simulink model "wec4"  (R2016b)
settings: Solver=ode4  StartTime=0  StopTime=1000  FixedStep=0.005  MaxStep=0.005  RelTol=1e-3  EnableMultiTasking=on
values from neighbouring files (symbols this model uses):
  arAdaptiveLawData = 1/2*zModelSimple.zModelPto.arFreq.*     zModelSimple.zModelPto.arMagnitude./     cos(zModelSimple.zModelPto.arPhase*pi/180+pi/2)    [IMPACT_Control.m]
  arAdaptiveLawDataX = 1/2*zModelSimpleX.zModelPto.arFreq.*         zModelSimpleX.zModelPto.arMagnitude./         cos(zModelSimpleX.zModelPto.arPhase*pi/180+pi/2)    [IMPACT_Control.m]
  arControllerRampGain = [0,0,1,1]    [IMPACT_Control.m]
  arControllerRampTime = [0 rStartRampTime rStartRampTime+rRampTimeLength 8000]    [IMPACT_Control.m]
  arEkfInitialisation = zeros(1,11)    [IMPACT_Control.m]
  arEkfInitialisationX = zeros(1,11)    [IMPACT_Control.m]
  arFrequency = zModelSimple.zModelPto.arFreq    [IMPACT_Control.m]
  arFrequencyRange = zModelSimple.zModelPto.arFreq    [IMPACT_Control.m]
  arFrequencyX = zModelSimpleX.zModelPto.arFreq    [IMPACT_Control.m]
  arImpedance = 1./zModelSimple.zModelPto.arMagnitude./zModelSimple.zModelPto.arFreq    [IMPACT_Control.m]
  arImpedanceX = 1./zModelSimpleX.zModelPto.arMagnitude./zModelSimpleX.zModelPto.arFreq    [IMPACT_Control.m]
  CentralPTOPreload = -1.6113e+07    (= -16113000)    [wecSimInputFile.m]
  F1 = [4.243 2.375 -12.243]    [wecSimInputFile.m]
  F2 = [4.243 -2.375 -12.243]    [wecSimInputFile.m]
  F3 = [-4.243 -2.375 -12.243]    [wecSimInputFile.m]
  F4 = [-4.243 2.375 -12.243]    [wecSimInputFile.m]
  FC = [0 0 -14]    [wecSimInputFile.m]
  iAdaptiveDamping = 0    [wec4IMPACT_Project.m]    (also in IMPACT_Control.m = handles.iAdaptiveDamping; wec1_IMPACT_Project.m; wec2_IMPACT_Project.m; wec3_IMPACT_Project.m)
  iControlType = 2    [wec4IMPACT_Project.m]    (also in IMPACT_Control.m = handles.iControlType; wec1_IMPACT_Project.m = 1; wec2_IMPACT_Project.m = 1; wec3_IMPACT_Project.m = 1)
  iPtoPositionConstraint = 1    [wec4IMPACT_Project.m]    (also in IMPACT_Control.m = handles.iPtoPositionConstraint; wec1_IMPACT_Project.m = 0; wec2_IMPACT_Project.m; wec3_IMPACT_Project.m)
  iSensorNoise = 0    [IMPACT_Control.m]
  m = m+1    (= 2)    [checkParamFile.m]
  PTOrotation = atan((T1(2)-F1(2))/(T1(1)-F1(1)))    [wecSimInputFile.m]
  rCogFloater = -8    [wec4_IMPACT_Model.m]    (also in paramInitial.m = get( handles.edit_rCogFloater, 'String' ); wec1_IMPACT_Model.m = -18; wec2_IMPACT_Model.m = -8.5; wec3_IMPACT_Model.m = -0.7)
  rCogSpar = -36.6    [wec4_IMPACT_Model.m]    (also in paramInitial.m = get( handles.edit_rCogSpar, 'String' ); wec3_IMPACT_Model.m = -21.3; wec3_IMPACT_Model2.m = -21.3)
  rDisplacementLimit = 10.000000    (= 10)    [wec4IMPACT_Project.m]    (also in IMPACT_Control.m = getValue(handles.edit_displacementLimit); wec1_IMPACT_Project.m; wec2_IMPACT_Project.m; wec3_IMPACT_Project.m = 3)
  rDisplacementLimitX = 10.000000    (= 10)    [wec4IMPACT_Project.m]    (also in IMPACT_Control.m = getValue(handles.edit_displacementLimitX); wec1_IMPACT_Project.m = 0; wec2_IMPACT_Project.m; wec3_IMPACT_Project.m = 0)
  rGainForAntiWIndUp = tfControllerDiscrete.rGain    [IMPACT_Control.m]
  rGainForAntiWIndUpX = tfControllerXDiscrete.rGain    [IMPACT_Control.m]
  rMaxForcePto = 300000000.000000    (= 300000000)    [wec4IMPACT_Project.m]    (also in IMPACT_Control.m = getValue(handles.edit_maxForcePto); wec1_IMPACT_Project.m = 1e+15; wec2_IMPACT_Project.m = 1e+15; wec3_IMPACT_Project.m = 1000000000)
  rMinForcePto = -300000000.000000    (= -300000000)    [wec4IMPACT_Project.m]    (also in IMPACT_Control.m = getValue(handles.edit_minForcePto); wec1_IMPACT_Project.m = -1e+15; wec2_IMPACT_Project.m = -1e+15; wec3_IMPACT_Project.m = -1000000000)
  rMooringX = 20000    [wec4_IMPACT_Model.m]    (also in paramInitial.m = get( handles.edit_rMooringX, 'String' ); wec3_IMPACT_Model.m = 10000; wec3_IMPACT_Model2.m = 10000)
  rMooringZ = 10000    [wec4_IMPACT_Model.m]    (also in paramInitial.m = get( handles.edit_rMooringZ, 'String' ); wec3_IMPACT_Model.m = 0; wec3_IMPACT_Model2.m = 0)
  rOutputSampleTime = 0.010000    (= 0.01)    [wec4IMPACT_Project.m]    (also in IMPACT_Control.m = getValue(handles.edit_outputSampleTime); wec1_IMPACT_Project.m; wec2_IMPACT_Project.m; wec3_IMPACT_Project.m)
  rPassiveDampingGain = -604830.000000    (= -604830)    [wec4IMPACT_Project.m]    (also in IMPACT_Control.m = getValue(handles.edit_gainPLD); wec1_IMPACT_Project.m = -214018.1537; wec2_IMPACT_Project.m = -1948070; wec3_IMPACT_Project.m = -519390)
  rPassiveDampingGainX = -278660.000000    (= -278660)    [wec4IMPACT_Project.m]    (also in IMPACT_Control.m = getValue(handles.edit_gainPLDX); wec1_IMPACT_Project.m = 0; wec2_IMPACT_Project.m = 0; wec3_IMPACT_Project.m = 0)
  rTetherPretension = 1.6113e+07    (= 16113000)    [wec4_IMPACT_Model.m]    (also in paramInitial.m = get( handles.edit_rTetherPretension, 'String' ); wec3_IMPACT_Model.m = 0; wec3_IMPACT_Model2.m = 0)
  rTetherSpring = 500000    [wec4_IMPACT_Model.m]    (also in paramInitial.m = get( handles.edit_rTetherSpring, 'String' ); wec3_IMPACT_Model.m = 0; wec3_IMPACT_Model2.m = 0)
  rUpperFrequencyLimit = EKFFloater.upperFreq    [IMPACT_Control.m]
  rXf = 4.243    [wec4AdditionalParams.m]
  rXs = 16.075    [wec4AdditionalParams.m]
  rYf = 2.375    [wec4AdditionalParams.m]
  rYs = 16.075    [wec4AdditionalParams.m]
  rZf = 4.243    [wec4AdditionalParams.m]
  rZs = 2.4350    (= 2.435)    [wec4AdditionalParams.m]
  rZTetherF = 6    [wec4AdditionalParams.m]
  rZTetherS = 2.4350    (= 2.435)    [wec4AdditionalParams.m]
  s = tf('s')    [wec4_IMPACT_Model.m]    (also in IMPACT_Control.m; wec1_IMPACT_Model.m; wec2_IMPACT_Model.m; wec3_IMPACT_Model.m)
  SidePTO1Preload = PreloadPTOCorner    (= 0)    [wecSimInputFile.m]
  SidePTO2Preload = PreloadPTOCorner    (= 0)    [wecSimInputFile.m]
  SidePTO3Preload = PreloadPTOCorner    (= 0)    [wecSimInputFile.m]
  SidePTO4Preload = PreloadPTOCorner    (= 0)    [wecSimInputFile.m]
  simu = simulationClass()    [wecSimInputFile.m]
  T1 = [16.075 16.075 -34.165]    [wecSimInputFile.m]
  T2 = [16.075 -16.075 -34.165]    [wecSimInputFile.m]
  T3 = [-16.075 -16.075 -34.165]    [wecSimInputFile.m]
  T4 = [-16.075 16.075 -34.165]    [wecSimInputFile.m]
  TC = [0 0 -34.165]    [wecSimInputFile.m]
  waves = waveClass('irregular')    [wecSimInputFile.m]
  Z = magPhaseToComplex(zModelTf)    [IMPACT_Control.m]
undefined symbols (not defined in the file or in its folder): arControllerDiscreteDen, arControllerDiscreteNum, arControllerDiscreteXDen, arControllerDiscreteXNum, arExcForceFloaterDen, arExcForceFloaterNum, arExcForceFloaterXDen, arExcForceFloaterXNum, arExcForceSparDen, arExcForceSparNum, arExcForceSparXDen, arExcForceSparXNum, arFexcFloaterDen, arFexcFloaterNum, arFexcFloaterXDen, arFexcFloaterXNum, arFexcSparDen, arFexcSparNum, arFexcSparXDen, arFexcSparXNum, Body, body, constraint, CTTime, deg, Elements, geometry, IRKB, kg, lenJ, mooring, N, pto, rAccelerationGainFloater, rAccelerationGainFloaterX, rAccelerationGainSpar, rAccelerationGainSparX, rad, rBuoyancyGainFloater, rBuoyancyGainFloaterX, rBuoyancyGainSpar, rBuoyancyGainSparX, rDampingGainFloater, rDampingGainFloaterX, rDampingGainSpar, rDampingGainSparX, Rigid, rMaxFocePto, wec4_float, wec4_reactor, WECSim_Lib, X, Y
libraries: nesl_utility x380, sm_lib x170, vrlib x91, simulink x12, WECSim_Lib x4
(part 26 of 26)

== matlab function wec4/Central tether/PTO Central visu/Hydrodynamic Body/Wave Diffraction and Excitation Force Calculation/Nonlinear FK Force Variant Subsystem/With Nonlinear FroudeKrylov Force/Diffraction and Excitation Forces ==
function [f, wp, wpMeanFS]  = nonFKForce(x,elv,center,tnorm,area,rho,g,cg,AH,w,dw,wDepth,deepWaterWave,k,typeNum,t,phaseRand)
% Function to calculate wave exitation force and moment on a triangulated surface
% NOTE: This function assumes that the STL file is imported with its CG at 0,0,0

% Logic to calculate nonFKForce at reduced sample time
[f, wp, wpMeanFS] = calc_force(x,elv,center,tnorm,area,rho,g,cg,AH,w,dw,wDepth,deepWaterWave,k,typeNum,t,phaseRand);
end

function [f, wp, wpMeanFS]  = calc_force(x,elv,center,tnorm,area,rho,g,cg,AH,w,dw,wDepth,deepWaterWave,k,typeNum,t,phaseRand)
% Function to apply translation and rotation, and calculate forces.

% Compute new tri coords after cog rotation and translation
centerMeanFS = offsetXYZ(center,cg);
avMeanFS     = tnorm .* [area area area];

% Compute new tri coords after cog rotation and translation
center = rotateXYZ(center,[1 0 0],x(4));
center = rotateXYZ(center,[0 1 0],x(5));
center = rotateXYZ(center,[0 0 1],x(6));
center = offsetXYZ(center,x);
center = offsetXYZ(center,cg);
% Compute new normal vectors coords after cog rotation and translation
tnorm = rotateXYZ(tnorm,[1 0 0],x(4));
tnorm = rotateXYZ(tnorm,[0 1 0],x(5));
tnorm = rotateXYZ(tnorm,[0 0 1],x(6));

% Copute area vectors
av = tnorm .* [area area area];

% Calculate the free surface
wpMeanFS=pDis(centerMeanFS,       0,AH,w,dw,wDepth,deepWaterWave,t,k,phaseRand,typeNum,rho,g);
wp      =pDis(center      ,     elv,AH,w,dw,wDepth,deepWaterWave,t,k,phaseRand,typeNum,rho,g);

% Calculate forces
f_linear   =FK(centerMeanFS,       cg,avMeanFS,wpMeanFS);
f_nonLinear=FK(center      ,x(1:3)+cg,av      ,wp      );
f = f_nonLinear-f_linear;
end

function verts = offsetXYZ(verts,x)
% Function to move the position vertices
verts(:,1) = verts(:,1) + x(1);
verts(:,2) = verts(:,2) + x(2);
verts(:,3) = verts(:,3) + x(3);
end

function xn = rotateXYZ(x,ax,t)
% Function to rotate a point about an arbitrary axis
% x: 3-componenet coordinates
% ax: axis about which to rotate (must be a vector length 1)
% t: rotation angle
% xn: new coordinates after rotation
rotMat = zeros(3);
rotMat(1,1) = ax(1)*ax(1)*(1-cos(t))    + cos(t);
rotMat(1,2) = ax(2)*ax(1)*(1-cos(t))    + ax(3)*sin(t);
rotMat(1,3) = ax(3)*ax(1)*(1-cos(t))    - ax(2)*sin(t);
rotMat(2,1) = ax(1)*ax(2)*(1-cos(t))    - ax(3)*sin(t);
rotMat(2,2) = ax(2)*ax(2)*(1-cos(t))    + cos(t);
rotMat(2,3) = ax(3)*ax(2)*(1-cos(t))    + ax(1)*sin(t);
rotMat(3,1) = ax(1)*ax(3)*(1-cos(t))    + ax(2)*sin(t);
rotMat(3,2) = ax(2)*ax(3)*(1-cos(t))    - ax(1)*sin(t);
rotMat(3,3) = ax(3)*ax(3)*(1-cos(t))    + cos(t);
xn = x*rotMat;
end

function f=pDis(center,elv,AH,w,dw,wDepth,deepWaterWave,t,k,phaseRand,typeNum,rho,g)
% Function to calculate pressure distribution
f = zeros(length(center(:,3)),1);
z=zeros(length(center(:,1)),1);
if typeNum <10
elseif typeNum <20
    f = rho.*g.*AH(1).*cos(k(1).*center(:,1)-w(1)*t);
    if deepWaterWave == 0
        z=(center(:,3)-elv).*wDepth./(wDepth+elv);
        f = f.*(cosh(k(1).*(z+wDepth))./cosh(k(1)*wDepth));
    else
        z=(center(:,3)-elv);
        f = f.*exp(k(1).*z);
    end
elseif typeNum <30
    for i=1:length(AH)
        if deepWaterWave == 0 && wDepth <= 0.5*pi/k(i)
            z=(center(:,3)-elv).*wDepth./(wDepth+elv);
            f_tmp = rho.*g.*sqrt(AH(i)*dw(i)).*cos(k(i).*center(:,1)-w(i)*t-phaseRand(i));
            f = f + f_tmp.*(cosh(k(i).*(z+wDepth))./cosh(k(i).*wDepth));
        else
            z=(center(:,3)-elv);
            f_tmp = rho.*g.*sqrt(AH(i)*dw(i)).*cos(k(i).*center(:,1)-w(i)*t-phaseRand(i));
            f = f + f_tmp.*exp(k(i).*z);
        end
    end
end
f(z>0)=0;
end

function f = FK(center,instcg,av,wp)
% Function to calculate the force and moment about the cog due to Froude-Krylov pressure
f = zeros(6,1);

% Calculate the hydrostatic pressure at each triangle center
pressureVect = [wp wp wp].*-av;

% Compute force about cog
f(1:3) = sum(pressureVect);

% Compute moment about cog
tmp1 = ones(length(center(:,1)),1);
tmp2 = tmp1*instcg';
center2cgVec = center-tmp2;

f(4:6)= sum(cross(center2cgVec,pressureVect));
end

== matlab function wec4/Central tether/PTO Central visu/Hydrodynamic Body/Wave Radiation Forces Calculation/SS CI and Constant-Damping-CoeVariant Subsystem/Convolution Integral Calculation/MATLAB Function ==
function F_FM = ConvolutionIntegral_interp(v, IRKB, lenJ, CTTime)
%#codegen
% Function to calculate convolution integral

%define persistent variables
interp_factor = 1;
persistent velocity IRKB_interp CTTime_interp;

if isempty(velocity) 
    CTTime_interp  = CTTime(1:interp_factor:end);
    velocity       = zeros(lenJ,length(CTTime_interp));
    IRKB_reordered = permute(IRKB,[3 1 2]);                     % permutes from [601 6 12] to [12 601 6]
    IRKB_interp    = IRKB_reordered(:,1:interp_factor:end, :);  % what does this do?
end 
% shift velocity
velocity      = circshift(velocity, 1, 2);
v = v(:)'';           %force v to be a column
velocity(:,1) = v(:);

%integrate
time_series = bsxfun(@times, IRKB_interp, velocity);
F_FM = squeeze(trapz(CTTime_interp,sum(time_series, 1)));

end

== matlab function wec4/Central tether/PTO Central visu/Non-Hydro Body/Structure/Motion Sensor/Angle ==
function E  = EulerAngle(Q)
% Euler Angle Type II or Tait-Bryan Angle for sequence 321 or zyx (Nautical or Cardan angles).
% Yaw [-180,180], followed by pitch [-90,90], followed by roll [-180,180]
E = zeros(3,1);
E(1) = atan2( (2*(Q(1)*Q(2)+Q(3)*Q(4))), (1-2* (Q(2)^2+Q(3)^2) ) );
E(2) = asin( 2* (Q(1)*Q(3) - Q(4)*Q(2)));
E(3) = atan2( (2*(Q(1)*Q(4)+Q(2)*Q(3))), (1-2* (Q(3)^2+Q(4)^2) ) );

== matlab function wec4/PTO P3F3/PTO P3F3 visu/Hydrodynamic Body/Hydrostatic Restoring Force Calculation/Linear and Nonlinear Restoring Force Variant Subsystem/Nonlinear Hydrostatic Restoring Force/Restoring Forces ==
function [f,p]  = nonLinearBuoyancy(x,elv,center,tnorm,area,rho,g,cg,mass)
% Function to calculate buoyancy force and moment on a triangulated surface
% NOTE: This function assumes that the STL file is imported with its CG at 0,0,0
[f,p] = calc_buoyancy(x,elv,center,tnorm,area,rho,g,cg);
f = -f + [0 0 g*mass 0 0 0]';
end


function [f,p] = calc_buoyancy(x,elv,center,tnorm,area,rho,g,cg)
% Function to apply translation and rotation and calculate forces

% Compute new tri coords after cog rotation and translation
center = rotateXYZ(center,[1 0 0],x(4));
center = rotateXYZ(center,[0 1 0],x(5));
center = rotateXYZ(center,[0 0 1],x(6));
center = offsetXYZ(center,x);
center = offsetXYZ(center,cg);
% Compute new normal vectors coords after cog rotation
tnorm = rotateXYZ(tnorm,[1 0 0],x(4));
tnorm = rotateXYZ(tnorm,[0 1 0],x(5));
tnorm = rotateXYZ(tnorm,[0 0 1],x(6));

% Calculate the hydrostatic forces
av = tnorm .* [area area area];
[f,p]=fHydrostatic(center,elv,x(1:3)+cg,av,rho,g);
end

function verts = offsetXYZ(verts,x)
% Function to move the position vertices
verts(:,1) = verts(:,1) + x(1);
verts(:,2) = verts(:,2) + x(2);
verts(:,3) = verts(:,3) + x(3);
end

function xn = rotateXYZ(x,ax,t)
% Function to rotate a point about an arbitrary axis
% x: 3-componenet coordiantes
% ax: axis about which to rotate (must be a vector length 1)
% t: rotation angle
% xn: new coordinates after rotation
rotMat = zeros(3);
rotMat(1,1) = ax(1)*ax(1)*(1-cos(t))    + cos(t);
rotMat(1,2) = ax(2)*ax(1)*(1-cos(t))    + ax(3)*sin(t);
rotMat(1,3) = ax(3)*ax(1)*(1-cos(t))    - ax(2)*sin(t);
rotMat(2,1) = ax(1)*ax(2)*(1-cos(t))    - ax(3)*sin(t);
rotMat(2,2) = ax(2)*ax(2)*(1-cos(t))    + cos(t);
rotMat(2,3) = ax(3)*ax(2)*(1-cos(t))    + ax(1)*sin(t);
rotMat(3,1) = ax(1)*ax(3)*(1-cos(t))    + ax(2)*sin(t);
rotMat(3,2) = ax(2)*ax(3)*(1-cos(t))    - ax(1)*sin(t);
rotMat(3,3) = ax(3)*ax(3)*(1-cos(t))    + cos(t);
xn = x*rotMat;
end

function [f,p] = fHydrostatic(center,elv,instcg,av,rho,g)
% Function to calculate the force and moment about the cog due to hydrostatic pressure
f = zeros(6,1);

% Zeor out regions above the mean free surface
z=center(:,3); z((z-elv)>0)=0;

% Calculate the hydrostatic pressure at each triangle center
pressureVect = rho*g.*[-z -z -z].*-av;
p = rho*g.*-z;
% Compute force about cog
f(1:3) = sum(pressureVect);

tmp1 = ones(length(center(:,1)),1);
tmp2 = tmp1*instcg';
center2cgVec = center-tmp2;

f(4:6)= sum(cross(center2cgVec,pressureVect));
end

== matlab function wec4/PTO P3F3/PTO P3F3 visu/Hydrodynamic Body/Morrison Element and ViscousDampingForceCalculation/Morrison Element Variant Subsystem/Morrison Element On/Irregular Wave 
Morison Force/MorrisonElements/MorisonElementIrregular/MATLAB Function ==
function [u,v,w,xa,ya,za] = calc_orbital_vel(disp, waveNumber, waveFreq, waveAmp, phase, time, rampT, waveDir, waterDepth, g)
%#codegen

[u,v,w,xa,ya,za] = orbital_velocity(disp, waveNumber, waveFreq, waveAmp, phase, time, rampT, waveDir, waterDepth, g);

== matlab function wec4/PTO P3F3/PTO P3F3 visu/Hydrodynamic Body/Morrison Element and ViscousDampingForceCalculation/Morrison Element Variant Subsystem/Morrison Element On/Regular Wave 
Morison Force/MorrisonElements/OrbitalVelocity/MATLAB Function ==
function [u,v,w,xa,ya,za] = calc_orbital_vel(disp, waveNumber, waveFreq, waveAmp, randPhase, time, rampT, waveDir, waterDepth, g)
%#codegen

[u,v,w,xa,ya,za] = orbital_velocity(disp, waveNumber, waveFreq, waveAmp, randPhase, time, rampT, waveDir, waterDepth, g);

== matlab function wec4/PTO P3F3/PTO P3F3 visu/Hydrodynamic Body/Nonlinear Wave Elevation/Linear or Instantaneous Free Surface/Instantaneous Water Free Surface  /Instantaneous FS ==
function f  = waveElevation(x,center,cg,AH,w,dw,k,typeNum,t,rampT,phaseRand,waveDir)
% Function to calculate the wave elevation at the ceontroids of triangulated surface
% NOTE: This function assumes that the STL file is imported with its CG at 0,0,0
f = calc_elev(x,center,cg,AH,w,dw,k,typeNum,t,rampT,phaseRand, waveDir);
end

function f = calc_elev(x,center,cg,AH,w,dw,k,typeNum,t,rampT,phaseRand,waveDir)
% Function to rotate and translate body and call wave elevation function at new locations

% Compute new tri center coords after cog rotation and translation
center = rotateXYZ(center,[1 0 0],x(4));
center = rotateXYZ(center,[0 1 0],x(5));
center = rotateXYZ(center,[0 0 1],x(6));
center = offsetXYZ(center,x);
center = offsetXYZ(center,cg);
% Calculate the free surface
f=waveElev(center,AH,w,dw,t,k,rampT,phaseRand,typeNum,waveDir);
end

function verts = offsetXYZ(verts,x)
% Function to move the position vertices
verts(:,1) = verts(:,1) + x(1);
verts(:,2) = verts(:,2) + x(2);
verts(:,3) = verts(:,3) + x(3);
end

function xn = rotateXYZ(x,ax,t)
% Function to rotate a point about an arbitrary axis
% x: 3-component coordinates
% ax: axis about which to rotate (must be a vector length 1)
% t: rotation angle
% xn: new coordinates after rotation
rotMat = zeros(3);
rotMat(1,1) = ax(1)*ax(1)*(1-cos(t))    + cos(t);
rotMat(1,2) = ax(2)*ax(1)*(1-cos(t))    + ax(3)*sin(t);
rotMat(1,3) = ax(3)*ax(1)*(1-cos(t))    - ax(2)*sin(t);
rotMat(2,1) = ax(1)*ax(2)*(1-cos(t))    - ax(3)*sin(t);
rotMat(2,2) = ax(2)*ax(2)*(1-cos(t))    + cos(t);
rotMat(2,3) = ax(3)*ax(2)*(1-cos(t))    + ax(1)*sin(t);
rotMat(3,1) = ax(1)*ax(3)*(1-cos(t))    + ax(2)*sin(t);
rotMat(3,2) = ax(2)*ax(3)*(1-cos(t))    - ax(1)*sin(t);
rotMat(3,3) = ax(3)*ax(3)*(1-cos(t))    + cos(t);
xn = x*rotMat;
end

function f=waveElev(center,AH,w,dw,t,k,rampT,phaseRand,typeNum,waveDir)
% Function to calculate the wave elevation at an array of points
f = zeros(length(center(:,3)),1);
cx = center(:,1);
cy = center(:,2);
X = cx*cos(waveDir*pi/180) + cy*sin(waveDir*pi/180);
if typeNum <10
elseif typeNum <20
    f = AH(1).*cos(k(1).*X-w(1)*t);
elseif typeNum <30
    tmp=sqrt(AH.*dw);
    tmp1 = ones(1,length(center(:,1)));
    tmp2 = (w.*t+phaseRand)*tmp1;
    tmp3 = cos(k*X'- tmp2);
    f(:,1) = tmp3'*tmp;
end
if t<=rampT
    rampF = (1+cos(pi+pi*t/rampT))/2;
    f = f.*rampF;
end
end

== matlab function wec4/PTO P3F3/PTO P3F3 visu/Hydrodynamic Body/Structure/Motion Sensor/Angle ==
function E  = EulerAngle(Q)
% Euler Angle Type II or Tait-Bryan Angle for sequence 321 or zyx (Nautical or Cardan angles).
% Yaw [-180,180], followed by pitch [-90,90], followed by roll [-180,180]
E = zeros(3,1);
E(1) = atan2((2*(Q(1)*Q(2)+Q(3)*Q(4))),(1-2*(Q(2)^2+Q(3)^2)));
E(2) = asin(2*(Q(1)*Q(3)-Q(4)*Q(2)));
E(3) = atan2((2*(Q(1)*Q(4)+Q(2)*Q(3))),(1-2*(Q(3)^2+Q(4)^2)));

== matlab function wec4/PTO P3F3/PTO P3F3 visu/Hydrodynamic Body/Wave Diffraction and Excitation Force Calculation/Linear Wave Excitation Force Variant Subsystem/Irregular Wave 
Excitation Force/MATLAB Function ==
function Fext = fcn(A,w,fExtRE,fExtIM,phaseRand,dw,time)
%#codegen

% persistent A1 B1 B11 C1 D1 D11 E1 E11

A1=bsxfun(@plus,w*time,pi/2);
B1= sin(bsxfun(@plus,A1,phaseRand));
B11 = sin(bsxfun(@plus,w*time,phaseRand));
C1 = sqrt(bsxfun(@times,A,dw));
D1 =bsxfun(@times,fExtRE,C1);
D11 = bsxfun(@times,fExtIM,C1);
E1 = bsxfun(@times,B1,D1);
E11 = bsxfun(@times,B11,D11);

Fext = sum(bsxfun(@minus,E1,E11));

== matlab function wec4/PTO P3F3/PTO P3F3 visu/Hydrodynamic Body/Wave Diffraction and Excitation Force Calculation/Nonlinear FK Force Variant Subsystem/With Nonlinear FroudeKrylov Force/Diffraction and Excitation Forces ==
function [f, wp, wpMeanFS]  = nonFKForce(x,elv,center,tnorm,area,rho,g,cg,AH,w,dw,wDepth,deepWaterWave,k,typeNum,t,phaseRand)
% Function to calculate wave exitation force and moment on a triangulated surface
% NOTE: This function assumes that the STL file is imported with its CG at 0,0,0

% Logic to calculate nonFKForce at reduced sample time
[f, wp, wpMeanFS] = calc_force(x,elv,center,tnorm,area,rho,g,cg,AH,w,dw,wDepth,deepWaterWave,k,typeNum,t,phaseRand);
end

function [f, wp, wpMeanFS]  = calc_force(x,elv,center,tnorm,area,rho,g,cg,AH,w,dw,wDepth,deepWaterWave,k,typeNum,t,phaseRand)
% Function to apply translation and rotation, and calculate forces.

% Compute new tri coords after cog rotation and translation
centerMeanFS = offsetXYZ(center,cg);
avMeanFS     = tnorm .* [area area area];

% Compute new tri coords after cog rotation and translation
center = rotateXYZ(center,[1 0 0],x(4));
center = rotateXYZ(center,[0 1 0],x(5));
center = rotateXYZ(center,[0 0 1],x(6));
center = offsetXYZ(center,x);
center = offsetXYZ(center,cg);
% Compute new normal vectors coords after cog rotation and translation
tnorm = rotateXYZ(tnorm,[1 0 0],x(4));
tnorm = rotateXYZ(tnorm,[0 1 0],x(5));
tnorm = rotateXYZ(tnorm,[0 0 1],x(6));

% Copute area vectors
av = tnorm .* [area area area];

% Calculate the free surface
wpMeanFS=pDis(centerMeanFS,       0,AH,w,dw,wDepth,deepWaterWave,t,k,phaseRand,typeNum,rho,g);
wp      =pDis(center      ,     elv,AH,w,dw,wDepth,deepWaterWave,t,k,phaseRand,typeNum,rho,g);

% Calculate forces
f_linear   =FK(centerMeanFS,       cg,avMeanFS,wpMeanFS);
f_nonLinear=FK(center      ,x(1:3)+cg,av      ,wp      );
f = f_nonLinear-f_linear;
end

function verts = offsetXYZ(verts,x)
% Function to move the position vertices
verts(:,1) = verts(:,1) + x(1);
verts(:,2) = verts(:,2) + x(2);
verts(:,3) = verts(:,3) + x(3);
end

function xn = rotateXYZ(x,ax,t)
% Function to rotate a point about an arbitrary axis
% x: 3-componenet coordinates
% ax: axis about which to rotate (must be a vector length 1)
% t: rotation angle
% xn: new coordinates after rotation
rotMat = zeros(3);
rotMat(1,1) = ax(1)*ax(1)*(1-cos(t))    + cos(t);
rotMat(1,2) = ax(2)*ax(1)*(1-cos(t))    + ax(3)*sin(t);
rotMat(1,3) = ax(3)*ax(1)*(1-cos(t))    - ax(2)*sin(t);
rotMat(2,1) = ax(1)*ax(2)*(1-cos(t))    - ax(3)*sin(t);
rotMat(2,2) = ax(2)*ax(2)*(1-cos(t))    + cos(t);
rotMat(2,3) = ax(3)*ax(2)*(1-cos(t))    + ax(1)*sin(t);
rotMat(3,1) = ax(1)*ax(3)*(1-cos(t))    + ax(2)*sin(t);
rotMat(3,2) = ax(2)*ax(3)*(1-cos(t))    - ax(1)*sin(t);
rotMat(3,3) = ax(3)*ax(3)*(1-cos(t))    + cos(t);
xn = x*rotMat;
end

function f=pDis(center,elv,AH,w,dw,wDepth,deepWaterWave,t,k,phaseRand,typeNum,rho,g)
% Function to calculate pressure distribution
f = zeros(length(center(:,3)),1);
z=zeros(length(center(:,1)),1);
if typeNum <10
elseif typeNum <20
    f = rho.*g.*AH(1).*cos(k(1).*center(:,1)-w(1)*t);
    if deepWaterWave == 0
        z=(center(:,3)-elv).*wDepth./(wDepth+elv);
        f = f.*(cosh(k(1).*(z+wDepth))./cosh(k(1)*wDepth));
    else
        z=(center(:,3)-elv);
        f = f.*exp(k(1).*z);
    end
elseif typeNum <30
    for i=1:length(AH)
        if deepWaterWave == 0 && wDepth <= 0.5*pi/k(i)
            z=(center(:,3)-elv).*wDepth./(wDepth+elv);
            f_tmp = rho.*g.*sqrt(AH(i)*dw(i)).*cos(k(i).*center(:,1)-w(i)*t-phaseRand(i));
            f = f + f_tmp.*(cosh(k(i).*(z+wDepth))./cosh(k(i).*wDepth));
        else
            z=(center(:,3)-elv);
            f_tmp = rho.*g.*sqrt(AH(i)*dw(i)).*cos(k(i).*center(:,1)-w(i)*t-phaseRand(i));
            f = f + f_tmp.*exp(k(i).*z);
        end
    end
end
f(z>0)=0;
end

function f = FK(center,instcg,av,wp)
% Function to calculate the force and moment about the cog due to Froude-Krylov pressure
f = zeros(6,1);

% Calculate the hydrostatic pressure at each triangle center
pressureVect = [wp wp wp].*-av;

% Compute force about cog
f(1:3) = sum(pressureVect);

% Compute moment about cog
tmp1 = ones(length(center(:,1)),1);
tmp2 = tmp1*instcg';
center2cgVec = center-tmp2;

f(4:6)= sum(cross(center2cgVec,pressureVect));
end

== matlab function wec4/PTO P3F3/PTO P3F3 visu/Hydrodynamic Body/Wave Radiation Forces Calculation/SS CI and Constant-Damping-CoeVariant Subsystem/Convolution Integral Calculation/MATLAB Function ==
function F_FM = ConvolutionIntegral_interp(v, IRKB, lenJ, CTTime)
%#codegen
% Function to calculate convolution integral

%define persistent variables
interp_factor = 1;
persistent velocity IRKB_interp CTTime_interp;

if isempty(velocity) 
    CTTime_interp  = CTTime(1:interp_factor:end);
    velocity       = zeros(lenJ,length(CTTime_interp));
    IRKB_reordered = permute(IRKB,[3 1 2]);                     % permutes from [601 6 12] to [12 601 6]
    IRKB_interp    = IRKB_reordered(:,1:interp_factor:end, :);  % what does this do?
end 
% shift velocity
velocity      = circshift(velocity, 1, 2);
v = v(:)'';           %force v to be a column
velocity(:,1) = v(:);

%integrate
time_series = bsxfun(@times, IRKB_interp, velocity);
F_FM = squeeze(trapz(CTTime_interp,sum(time_series, 1)));

end

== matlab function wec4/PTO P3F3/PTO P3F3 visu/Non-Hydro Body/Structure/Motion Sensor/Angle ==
function E  = EulerAngle(Q)
% Euler Angle Type II or Tait-Bryan Angle for sequence 321 or zyx (Nautical or Cardan angles).
% Yaw [-180,180], followed by pitch [-90,90], followed by roll [-180,180]
E = zeros(3,1);
E(1) = atan2( (2*(Q(1)*Q(2)+Q(3)*Q(4))), (1-2* (Q(2)^2+Q(3)^2) ) );
E(2) = asin( 2* (Q(1)*Q(3) - Q(4)*Q(2)));
E(3) = atan2( (2*(Q(1)*Q(4)+Q(2)*Q(3))), (1-2* (Q(3)^2+Q(4)^2) ) );
